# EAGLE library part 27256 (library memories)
EPROM 32K x 8 bits
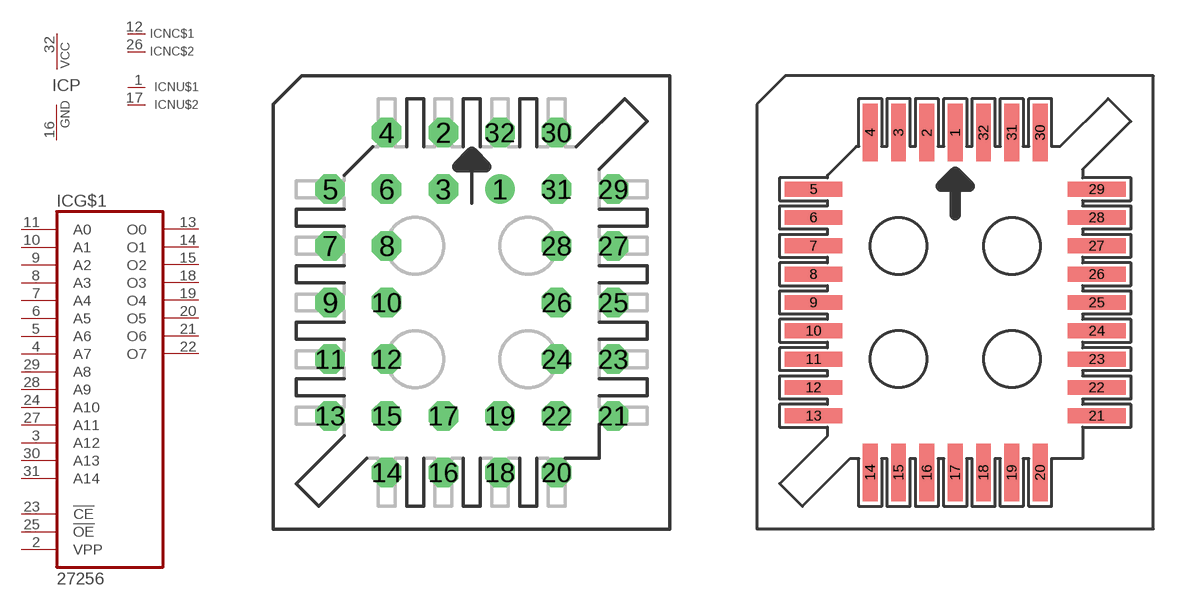
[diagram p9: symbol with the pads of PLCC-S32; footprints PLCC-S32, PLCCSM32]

Designator prefix IC; gates G$1=27256 P=PWRN NC$1=NC NC$2=NC NU$1=NU NU$2=NU

## 27256S  [PLCC-S32]
1  NU$1:IC-NU  nc
2  G$1:VPP  in
3  G$1:A12  in
4  G$1:A7  in
5  G$1:A6  in
6  G$1:A5  in
7  G$1:A4  in
8  G$1:A3  in
9  G$1:A2  in
10  G$1:A1  in
11  G$1:A0  in
12  NC$1:NC  nc
13  G$1:O0  hiz
14  G$1:O1  hiz
15  G$1:O2  hiz
16  P:GND  pwr
17  NU$2:IC-NU  nc
18  G$1:O3  hiz
19  G$1:O4  hiz
20  G$1:O5  hiz
21  G$1:O6  hiz
22  G$1:O7  hiz
23  G$1:!CE  in
24  G$1:A10  in
25  G$1:!OE  in
26  NC$2:NC  nc
27  G$1:A11  in
28  G$1:A9  in
29  G$1:A8  in
30  G$1:A13  in
31  G$1:A14  in
32  P:VCC  pwr

## 27256SMT  [PLCCSM32]
Pads as for PLCC-S32

## Footprint PLCC-S32 (pad centres in mm)
Plastic Leaded Chip Carrier Socket
drill 0.813: 1 1.27,5.08
drill 0.813 octagon: 2 -1.27,7.62; 3 -1.27,5.08; 4 -3.81,7.62; 5 -6.35,5.08; 6 -3.81,5.08; 7 -6.35,2.54; 8 -3.81,2.54; 9 -6.35,0; 10 -3.81,0; 11 -6.35,-2.54; 12 -3.81,-2.54; 13 -6.35,-5.08; 14 -3.81,-7.62; 15 -3.81,-5.08; 16 -1.27,-7.62; 17 -1.27,-5.08; 18 1.27,-7.62; 19 1.27,-5.08; 20 3.81,-7.62; 21 6.35,-5.08; 22 3.81,-5.08; 23 6.35,-2.54; 24 3.81,-2.54; 25 6.35,0; 26 3.81,0; 27 6.35,2.54; 28 3.81,2.54; 29 6.35,5.08; 30 3.81,7.62; 31 3.81,5.08; 32 1.27,7.62

## Footprint PLCCSM32 (pad centres in mm)
smd 0.66 x 2.591: 1 0,7.62; 2 -1.27,7.62; 3 -2.54,7.62; 4 -3.81,7.62; 14 -3.81,-7.62; 15 -2.54,-7.62; 16 -1.27,-7.62; 17 0,-7.62; 18 1.27,-7.62; 19 2.54,-7.62; 20 3.81,-7.62; 30 3.81,7.62; 31 2.54,7.62; 32 1.27,7.62
smd 2.591 x 0.66: 5 -6.35,5.08; 6 -6.35,3.81; 7 -6.35,2.54; 8 -6.35,1.27; 9 -6.35,0; 10 -6.35,-1.27; 11 -6.35,-2.54; 12 -6.35,-3.81; 13 -6.35,-5.08; 21 6.35,-5.08; 22 6.35,-3.81; 23 6.35,-2.54; 24 6.35,-1.27; 25 6.35,0; 26 6.35,1.27; 27 6.35,2.54; 28 6.35,3.81; 29 6.35,5.08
